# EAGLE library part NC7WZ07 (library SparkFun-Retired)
Ultra-high speed dual open-drain output buffer (non-inverting) Retired: IC-09351
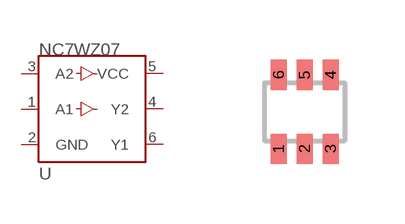
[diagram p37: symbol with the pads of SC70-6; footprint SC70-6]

Designator prefix -

## NC7WZ07  [SC70-6]
1  A1
2  GND
3  A2
4  Y2
5  VCC
6  Y1

## Footprint SC70-6 (pad centres in mm)
smd 0.4 x 0.75: 1 -0.65,-0.925; 2 0,-0.925; 3 0.65,-0.925; 4 0.65,0.925; 5 0,0.925; 6 -0.65,0.925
